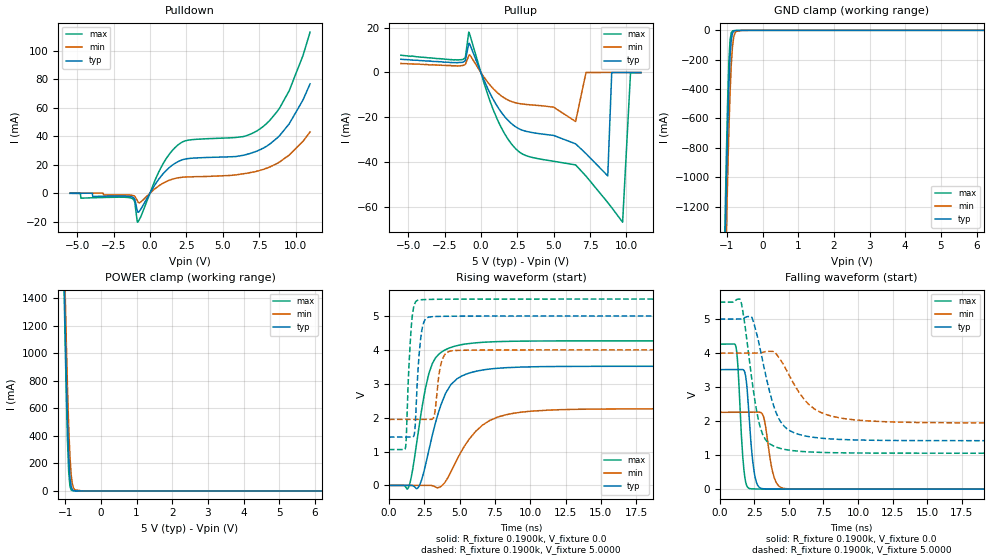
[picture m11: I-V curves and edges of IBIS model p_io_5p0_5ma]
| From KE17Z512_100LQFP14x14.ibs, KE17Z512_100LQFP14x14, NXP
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[Model] p_io_5p0_5ma
|   Model p_io_5p0_5ma
| This model was characterised for following simulation conditions:
| External (pad) voltage:
|   - Typ: 5.0V,   - Min: 4.0V,   - Max: 5.5V
| Library cells for typ/min/max conditions are connected as defined below:
|  pad - External Pad
|  ipp_do_lv - Core Input
|  ipp_obe_lv - Output Buffer Enable
|  abt_close_nor_rst_mv - vdde
|  dvdd - dvdd
|  dvss - dvss
|  esd_boost - vdde
|  ipp_ina_280_mv - NC
|  ipp_ina_40_a_mv - NC
|  ipp_ina_40_b_mv - NC
|  ipp_ina_40_c_mv - NC
|  ipp_ina_40_d_mv - NC
|  ipp_ina_40_e_mv - NC
|  ipp_ina_40_f_mv - NC
|  ipp_ina_40_g_mv - NC
|  ipp_ina_40_h_mv - NC
|  ipp_ind_lv - NC
|  vdde - vdde
|  vsse - vsse
| All other pins connected to ground
Model_type I/O
Polarity   Non-Inverting
Enable   Active-High
Vinl =   1.5000V
Vinh =   3.5000V
Vmeas =  2.5000V
Cref =   50.0000F
C_comp   1.4688pF   1.4069pF   1.5565pF
[Model Spec]
| variable   typ   min   max
Vinh   3.5000V   2.8000V   3.8500V
Vinl   1.5000V   1.2000V   1.6500V
S_overshoot_high   5.3000V   4.3000V   5.8000V
S_overshoot_low   -0.3000V   -0.3000V   -0.3000V
Vmeas   2.5000V   2.0000V   2.7500V
[Temperature Range]   25.0000   0.1250k   -40.0000
[Voltage Range]   5.0000V   4.0000V   5.5000V
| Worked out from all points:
|   slope of the pulldown table from 0 to 0.75 V, typ, clamps not added: 63.5 ohm
|   slope of the pullup table from 0 to 0.75 V, typ, clamps not added: 69.2 ohm
|   GND clamp passes 1 mA (typ) near -0.71 V on its own axis
|   POWER clamp passes 1 mA (typ) near -0.73 V on its own axis
|   rising waveform, R_fixture 0.1900k, V_fixture 0.0: 20-80 % time 1.5ns typ, 2.28ns min, 1.09ns max; typ from 0 V to 3.52 V
|   rising waveform, R_fixture 0.1900k, V_fixture 5.0000: 20-80 % time 326ps typ, 376ps min, 297ps max; typ from 1.43 V to 5 V
|   falling waveform, R_fixture 0.1900k, V_fixture 0.0: 20-80 % time 417ps typ, 533ps min, 340ps max; typ from 3.52 V to 0 V
|   falling waveform, R_fixture 0.1900k, V_fixture 5.0000: 20-80 % time 1.36ns typ, 2.15ns min, 957ps max; typ from 5 V to 1.43 V
[Pulldown]
|Voltage   I(typ)   I(min)   I(max)
-5.5V     -20uA      10uA       -150uA
-4.786V   -10uA      0A         -260uA
-4.752V   -20uA      0A         -3.5mA
-1.25V    -2.592mA   -1.452mA   -3.606mA
-1.046V   -4.395mA   -2.22mA    -6.539mA
-842mV    -13.31mA   -5.887mA   -20.36mA
756mV     11.88mA    6.141mA    18.04mA
1.946V    22.23mA    10.81mA    34.02mA
6.604V    27.1mA     13.9mA     40.23mA
8.236V    34.5mA     18.4mA     51.1mA
9.562V    48.6mA     26.7mA     71.8mA
11V       76.7mA     42.9mA     113mA
[Pullup]
|Voltage   I(typ)   I(min)   I(max)
-5.5V     5.9mA      4mA        7.7mA
-1.24V    4.54mA     3.1mA      5.77mA
-832mV    12.96mA    7.49mA     18.05mA
834mV     -11.89mA   -7.151mA   -16.41mA
2.16V     -23.18mA   -13.13mA   -32.42mA
6.512V    -31.92mA   -21.93mA   -41.34mA
7.226V    -36.29mA   -10uA      -46.35mA
8.722V    -46.25mA   10uA       -58.17mA
8.994V    -40uA      10uA       -60.45mA
9.742V    -10uA      0A         -66.95mA
10.29V    -20uA      0A         -180uA
11V       -30uA      -10uA      -140uA
[GND_clamp]
|Voltage   I(typ)   I(min)   I(max)
-5.5V     -69.44A    -69.33A    -69.56A
-1.08V    -1.862A    -2.181A    -1.676A
-1.046V   -1.439A    -1.766A    -1.242A
-1.012V   -1.042A    -1.375A    -839mA
-978mV    -685.9mA   -1.014A    -486.5mA
-944mV    -390.5mA   -694.3mA   -218.1mA
-910mV    -180.5mA   -430mA     -67.94mA
-876mV    -65.97mA   -234.5mA   -16.33mA
-842mV    -20.61mA   -111.6mA   -4.471mA
-774mV    -2.315mA   -19.16mA   -1.535mA
-570mV    -202.3uA   -200.8uA   -318.9uA
11V       0A         0A         0A
[POWER_clamp]
|Voltage   I(typ)   I(min)   I(max)
-5.5V     74.04A     73.75A     74.28A
-1.036V   1.665A     1.884A     1.547A
-1.002V   1.234A     1.468A     1.101A
-968mV    840.5mA    1.084A     696.4mA
-934mV    503.4mA    742.9mA    360.4mA
-900mV    248.8mA    460.3mA    134.4mA
-866mV    96.41mA    250.6mA    34.26mA
-832mV    30.4mA     118.7mA    7.218mA
-798mV    8.721mA    50.13mA    1.674mA
-730mV    840.9uA    7.627mA    381.1uA
-526mV    31.96uA    66.96uA    28.29uA
11V       0A         0A         0A
[Ramp]
| variable   typ   min   max
dV/dt_r  2.1095/1.4979n   1.3562/2.2791n   2.5595/1.0905n
dV/dt_f  2.1448/1.3552n   1.2322/2.1454n   2.6656/0.9568n
R_load = 0.1900k
[Rising Waveform]
R_fixture= 0.1900k
V_fixture= 0.0
V_fixture_min= 0.0
V_fixture_max= 0.0
|time   V(typ)   V(min)   V(max)
0s        1.011nV    12.16nV    7.41nV
1.376ns   -16.11uV   -11.22uV   -74.3mV
2.112ns   -41.25mV   -618.3nV   1.674V
2.599ns   610.1mV    -4.343uV   2.885V
3.054ns   1.447V     -7.108mV   3.58V
3.689ns   2.385V     -28.52mV   3.924V
4.548ns   3.039V     529.7mV    4.097V
6.602ns   3.403V     1.771V     4.224V
9.405ns   3.493V     2.163V     4.259V
40ns      3.516V     2.26V      4.266V
[Rising Waveform]
R_fixture= 0.1900k
V_fixture= 5.0000
V_fixture_min= 4.0000
V_fixture_max= 5.5000
|time   V(typ)   V(min)   V(max)
0s        1.425V     1.946V     1.057V
1.182ns   1.425V     1.946V     1.128V
1.626ns   1.425V     1.946V     4.881V
1.837ns   1.617V     1.946V     5.373V
2.1ns     3.637V     1.946V     5.471V
2.614ns   4.918V     1.947V     5.487V
3.228ns   4.984V     2.09V      5.493V
3.808ns   4.991V     3.746V     5.496V
4.528ns   4.995V     3.975V     5.497V
40ns      5V         4V         5.5V
[Falling Waveform]
R_fixture= 0.1900k
V_fixture= 0.0
V_fixture_min= 0.0
V_fixture_max= 0.0
|time   V(typ)   V(min)   V(max)
0s        3.516V     2.26V      4.266V
1.186ns   3.515V     2.26V      4.165V
1.725ns   3.507V     2.26V      669.3mV
1.943ns   3.114V     2.26V      113.8mV
2.162ns   1.906V     2.26V      17.26mV
2.745ns   112.1mV    2.263V     4.347mV
3.208ns   10.37mV    2.072V     2.582mV
3.938ns   3.657mV    344.6mV    1.429mV
4.724ns   1.927mV    16.64mV    863.8uV
40ns      140.3nV    352.4nV    74.94nV
[Falling Waveform]
R_fixture= 0.1900k
V_fixture= 5.0000
V_fixture_min= 4.0000
V_fixture_max= 5.5000
|time   V(typ)   V(min)   V(max)
0s        5V         4V         5.5V
1.502ns   4.999V     4V         5.561V
2.323ns   5.049V     4V         3.229V
2.692ns   4.543V     3.999V     2.254V
3.084ns   3.816V     4.022V     1.63V
3.768ns   2.625V     4.053V     1.295V
4.326ns   2.037V     3.84V      1.203V
6.436ns   1.546V     2.494V     1.095V
9.146ns   1.456V     2.067V     1.067V
40ns      1.425V     1.946V     1.057V
